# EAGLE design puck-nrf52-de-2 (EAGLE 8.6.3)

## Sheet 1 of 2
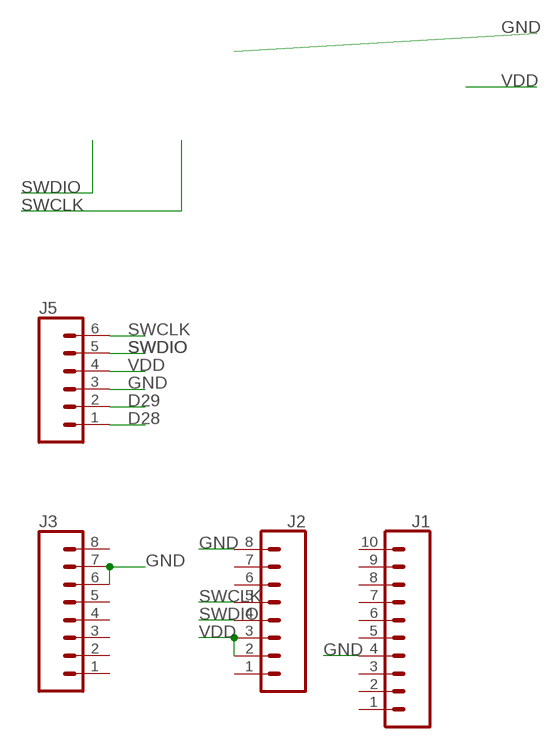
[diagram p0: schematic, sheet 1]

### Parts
J1  CONN_10"  [1X10]
J2  CONN_08"  [1X08]
J3  CONN_08"  [1X08]
J5  CONN_06SILK_FEMALE_PTH  [1X06]

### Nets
D28: J5.1 ; also sheet 2
D29: J5.2 ; also sheet 2
GND: J1.4 J2.8 J3.6 J3.7 J5.3
SWCLK: J2.5 J5.6 ; also sheet 2
SWDIO: J2.4 J5.5 ; also sheet 2
VDD: J2.2 J2.3 J5.4
Unconnected: J1.1 J1.2 J1.3 J1.5 J1.6 J1.7 J1.8 J1.9 J1.10 J2.1 J2.6 J2.7 J3.1 J3.2 J3.3 J3.4 J3.5 J3.8

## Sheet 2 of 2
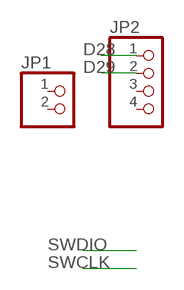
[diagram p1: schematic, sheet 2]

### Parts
JP1  PINHD-1X2  [1X02]
JP2  PINHD-1X4  [1X04]

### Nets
D28: JP2.1 ; also sheet 1
D29: JP2.2 ; also sheet 1
Unconnected: JP1.1 JP1.2 JP2.3 JP2.4

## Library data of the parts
J1 = SparkFun-Connectors:CONN_10: Multi connection point. Often used as Generic Header-pin footprint for 0.1 inch spaced/style header connections On any of the 0.1 inch spaced packages, you can populate with these: Break Away Headers - Straight (PRT-00116) Break Away Male Headers - Right Angle (PRT-00553) Female Headers (PRT-00115)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; PROD_ID: CONN-11563
J2 J3 = SparkFun-Connectors:CONN_08: Multi connection point. Often used as Generic Header-pin footprint for 0.1 inch spaced/style header connections On any of the 0.1 inch spaced packages, you can populate with these: Break Away Headers - Straight (PRT-00116) Break Away Male Headers - Right Angle (PRT-00553) Female Headers (PRT-00115)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; PROD_ID: CONN-08438
J5 = SparkFun-Connectors:CONN_06: Multi connection point. Often used as Generic Header-pin footprint for 0.1 inch spaced/style header connections On any of the 0.1 inch spaced packages, you can populate with these: Break Away Headers - Straight (PRT-00116) Break Away Male Headers - Right Angle (PRT-00553) Female Headers (PRT-00115)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; PROD_ID: CONN-08437
JP1 = pinhead:PINHD-1X2: PIN HEADER
JP2 = pinhead:PINHD-1X4: PIN HEADER

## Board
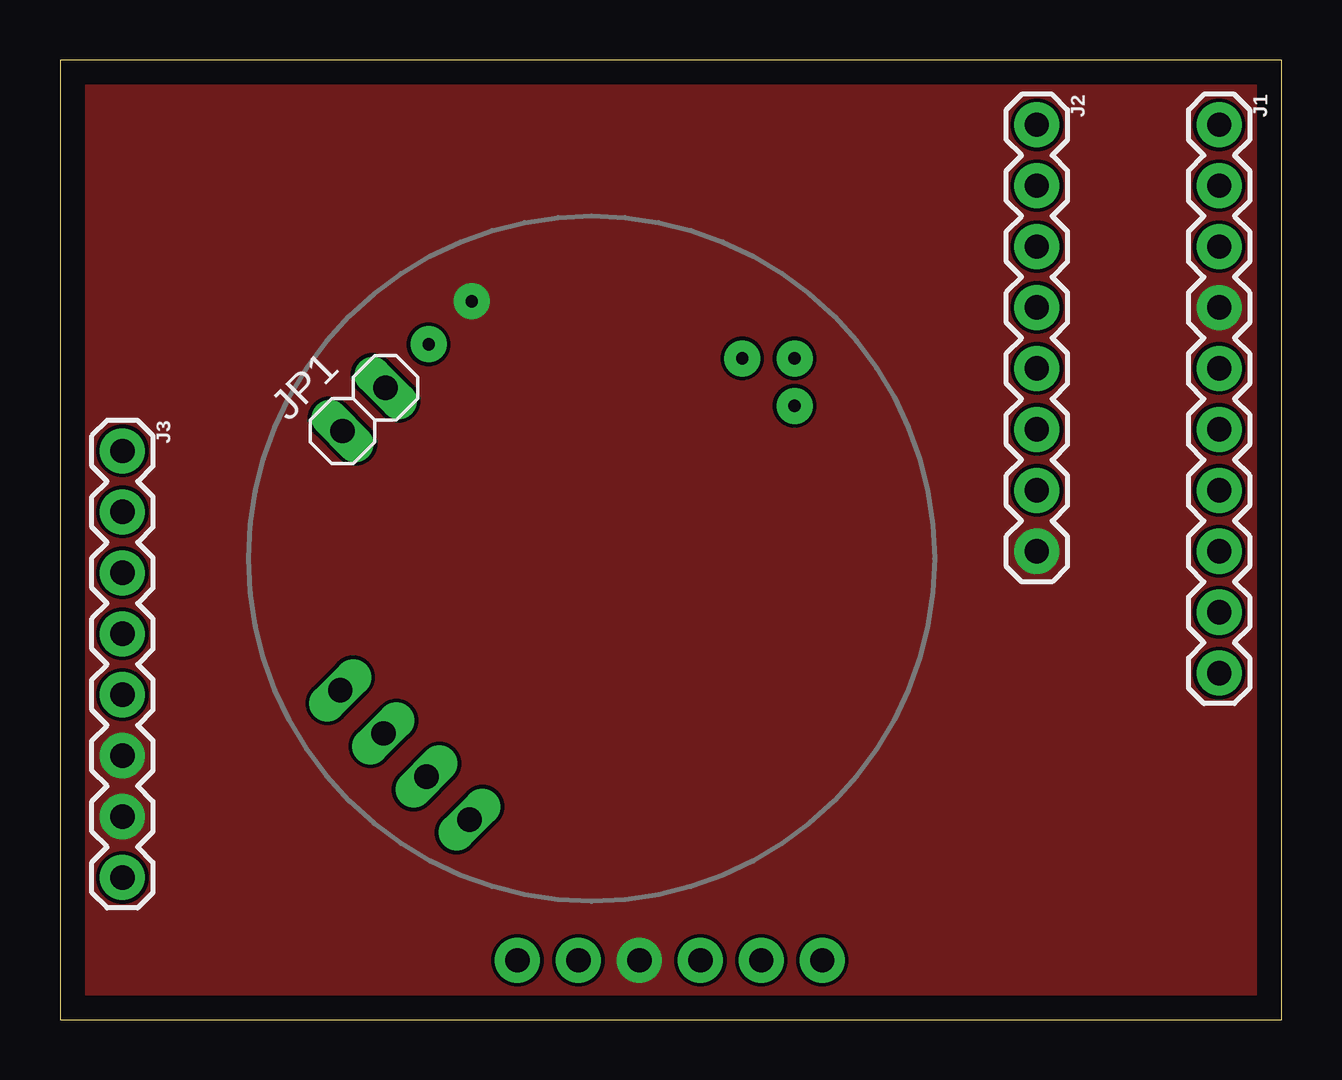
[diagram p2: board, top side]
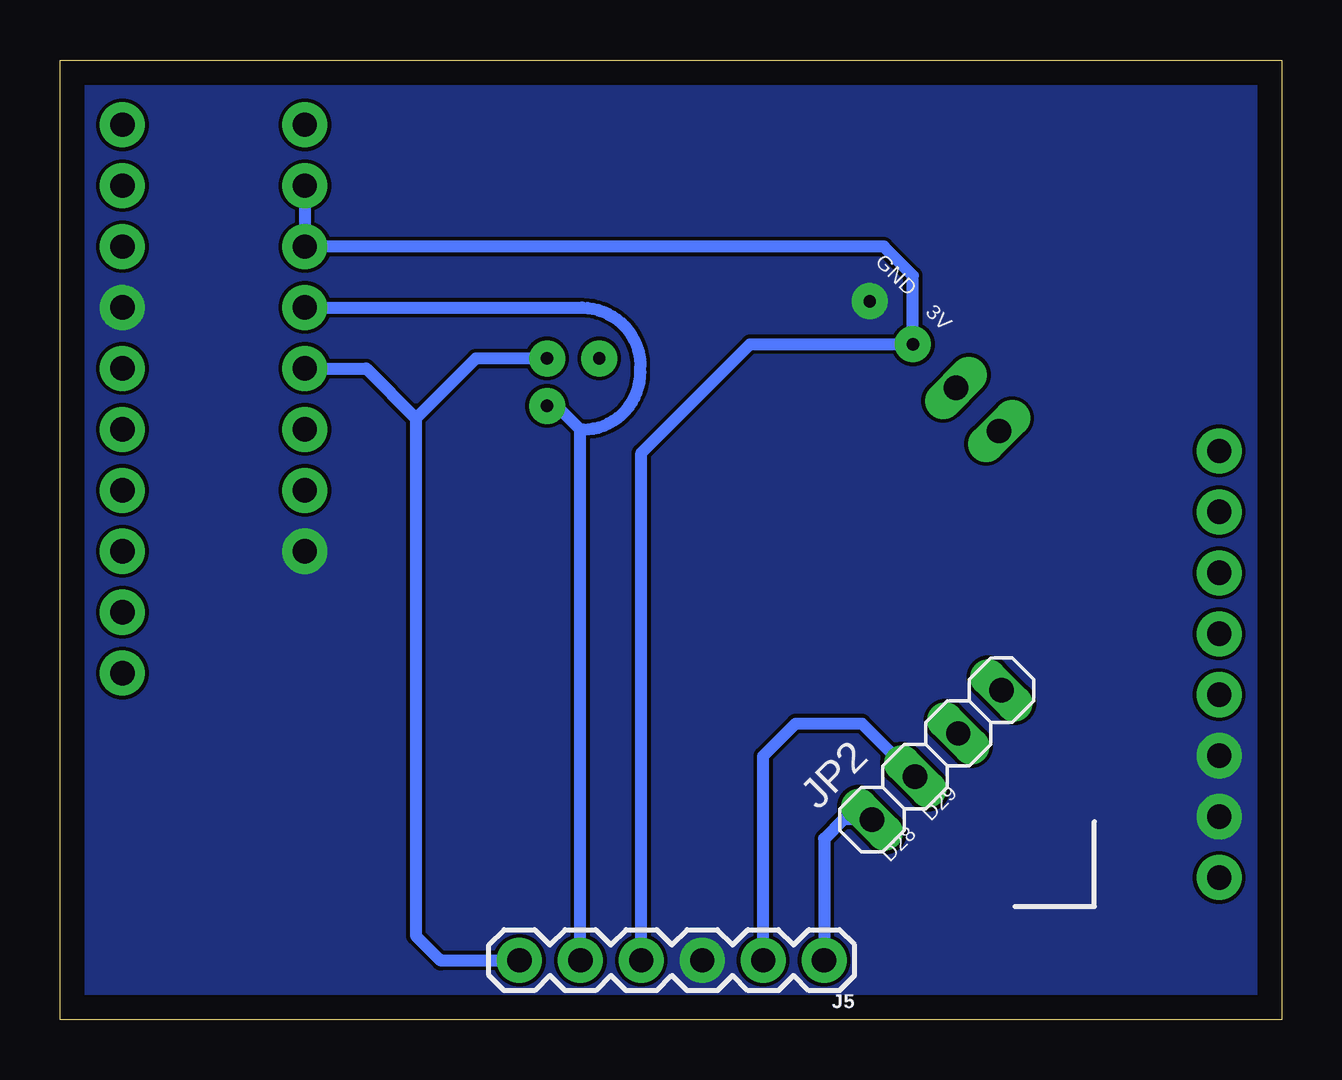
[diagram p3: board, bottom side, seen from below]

Size 50.9 x 40 mm. Coordinates in mm from the lower left corner, seen from the top.
Outline: 0,0 50.9,0 50.9,40 0,40 0,0
Copper layers (1*16): Top 0.035mm / dielectric 1.5mm / Bottom 0.035mm
Design rules "default": minimum track width 6mil, minimum drill 0.35mm, track to track 6mil, track to pad 6mil, pad to pad 6mil, via to via 6mil, smd to smd 6mil, copper to edge 40mil, drill to drill 6mil, minimum pad ring 10mil, minimum via ring 8mil, stop-mask expansion 4mil, vias tented up to drill 0mil, thermal gap 10mil

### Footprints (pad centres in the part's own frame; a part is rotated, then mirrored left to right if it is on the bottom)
1X10 = drill 1.016 pad 1.88: 1 0,0; 2 2.54,0; 3 5.08,0; 4 7.62,0; 5 10.16,0; 6 12.7,0; 7 15.24,0; 8 17.78,0; 9 20.32,0; 10 22.86,0
1X08 = drill 1.016 pad 1.88: 1 0,0; 2 2.54,0; 3 5.08,0; 4 7.62,0; 5 10.16,0; 6 12.7,0; 7 15.24,0; 8 17.78,0
1X06 = drill 1.016 pad 1.88: 1 0,0; 2 2.54,0; 3 5.08,0; 4 7.62,0; 5 10.16,0; 6 12.7,0
1X02 = drill 1.016 long: 1 -1.27,0; 2 1.27,0
1X04 = drill 1.016 long: 1 -3.81,0; 2 -1.27,0; 3 1.27,0; 4 3.81,0

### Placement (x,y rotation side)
J1  48.3,37.3 270 top
J2  40.7,37.3 270 top
J3  2.6,23.7 270 top
J5  19.06,2.47 180 bottom
JP1  12.67,25.43 45 top
JP2  14.37,11.03 45 bottom

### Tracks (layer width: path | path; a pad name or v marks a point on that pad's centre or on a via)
D28
  Bottom 0.508: JP2.1 18.26,8.34 19.06,7.54 J5.1
D29
  Bottom 0.508: J5.2 21.6,10.98 20.24,12.34 17.49,12.34 15.28,10.13 JP2.2
GND  (via drill 0.51 pad 1.5)
  other vias: 17.16,29.94
  pour Bottom (no thermals): 51.08,-0.2 51.08,40.21 -0.2,40.21 -0.2,-0.2
  pour Top (no thermals): 51.08,-0.2 51.08,40.21 -0.2,40.21 -0.2,-0.2
RESET  (via drill 0.51 pad 1.5)
  other vias: 28.43,27.56
SWCLK  (via drill 0.51 pad 1.5)
  Bottom 0.508: v30.61,27.56 33.57,27.56 36.07,25.06 | 36.07,25.06 36.07,3.49 35.03,2.45 35.01,2.47 J5.6 | J2.5 38.15,27.14 36.07,25.06
SWDIO  (via drill 0.51 pad 1.5)
  Bottom 0.508: J5.5 29.22,24.6 | 29.22,24.6 29.1,24.6 arc-90 26.72,26.98 26.72,27.24 arc-90 29.15,29.67 29.16,29.68 J2.4 | v30.61,25.58 30.21,25.58 29.22,24.6
VDD  (via drill 0.51 pad 1.5)
  Bottom 0.508: J2.2 J2.3 16.57,32.22 15.36,31.01 v15.36,28.15 22.15,28.15 26.68,23.62 J5.4

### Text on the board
bNames: GND | 3V | D29 | D28
tStop: Puck.js Programmer
bStop: LINE Things / Programmer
